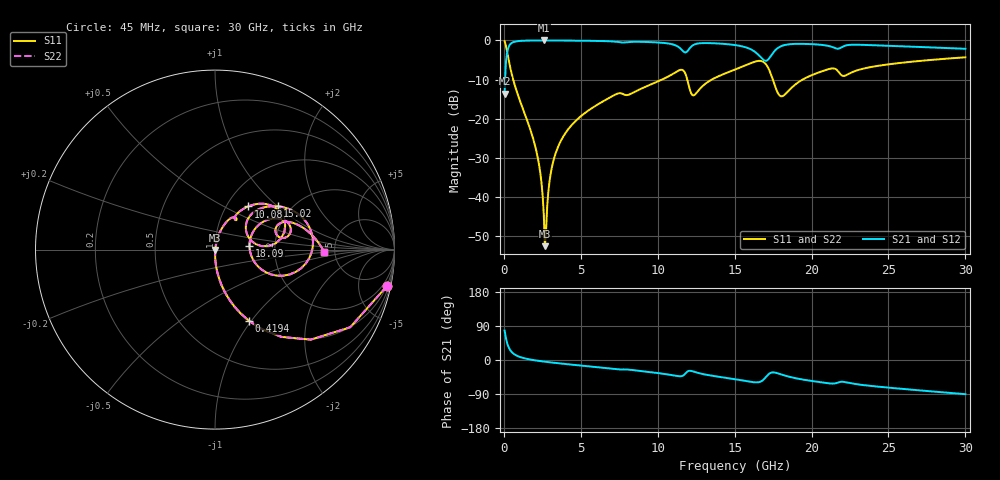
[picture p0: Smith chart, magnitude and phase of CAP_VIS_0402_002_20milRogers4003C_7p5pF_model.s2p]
! S-parameter model data by Modelithics Inc.  support@modelithics.com  813-866-6335  Tampa FL USA
! S-Parameter data specifications:
! Substrate: 20-mil Rogers 4003C, substrate thickness, H=0.508mm, Dielectric constant, Er=3.75
! PCB Mounting Pad Footprint: Pad width, PadW=0.50mm , Pad length, PadL=0.50mm , Pad gap, PadG (edge-to-edge)=0.40mm , Reference planes=1.4mm apart
! Created Wed Nov 18 12:49:41 2015
# hz S ma R 50
! 2 Port Network Data from SP1.SP block
! freq  magS11  angS11  magS21  angS21  magS12  angS12  magS22  angS22
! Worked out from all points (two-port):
!   401 points, 45 MHz to 30 GHz, reference 50 ohm
!   highest |S21| = -0.02 dB at 2.591 GHz (marker M1); lowest = -13.6 dB at 45 MHz (marker M2)
!   |S21| within 3 dB of the highest: 213.5 MHz to 11.73 GHz (11.52 GHz wide, 193 % of centre); 17.53 GHz to end of sweep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
!   lowest |S11| = -52.6 dB at 2.666 GHz (marker M3), VSWR 1.00, Z = 50.2 - j0.135 ohm
!   |S11| at or under -10 dB: 601 MHz to 10.28 GHz (9.682 GHz wide, 178 % of centre); 11.92 GHz to 13.52 GHz (1.603 GHz wide, 12.6 % of centre); 17.48 GHz to 19.43 GHz (1.946 GHz wide, 10.5 % of centre)
!   |S22| runs from -52.6 to -0.2 dB; largest |S21 - S12| = 0
!   S11 on the Smith chart (normalised r, x): 45 MHz: 0.99, -9.31; 419.4 MHz: 0.99, -0.97; 10.08 GHz: 1.26, +0.67; 15.02 GHz: 1.70, +1.00; 18.09 GHz: 1.47, +0.07; 30 GHz: 4.10, -0.17
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4.5e7  0.9779 -12.1  0.2089 77.9  0.2089 77.9  0.9779 -12.1
2.696625e8  0.6117 -52.7  0.7905 37.3  0.7905 37.3  0.6117 -52.7
4.194375e8  0.44 -64.5  0.8972 25.4  0.8972 25.4  0.44 -64.5
8.687625e8  0.2122 -78.9  0.976 10.8  0.976 10.8  0.2122 -78.9
2.066962e9  0.04177 -88.7  0.9973 -1.1  0.9973 -1.1  0.04177 -88.7
2.366512e9  0.02014 -87.5  0.9978 -2.9  0.9978 -2.9  0.02014 -87.5
2.591175e9  0.006033 -74.7  0.9979 -4.1  0.9979 -4.1  0.006033 -74.7
2.666062e9  0.00235 -34.8  0.9979 -4.5  0.9979 -4.5  0.00235 -34.8
2.815838e9  0.007757 69.2  0.9978 -5.2  0.9978 -5.2  0.007757 69.2
3.0405e9  0.01983 77.4  0.9975 -6.3  0.9975 -6.3  0.01983 77.4
3.414938e9  0.03864 78.5  0.9968 -8.0  0.9968 -8.0  0.03864 78.5
5.062462e9  0.1098 73.4  0.9907 -14.9  0.9907 -14.9  0.1098 73.4
1.007992e10  0.3033 52.4  0.9383 -34.8  0.9383 -34.8  0.3033 52.4
1.157768e10  0.4208 23.6  0.7517 -42.4  0.7517 -42.4  0.4208 23.6
1.232655e10  0.1979 25.5  0.8753 -30.5  0.8753 -30.5  0.1979 25.5
1.50225e10  0.424 34.7  0.8713 -50.7  0.8713 -50.7  0.424 34.7
1.68198e10  0.5376 -1.9  0.5739 -53.8  0.5739 -53.8  0.5376 -1.9
1.734401e10  0.3755 -22.7  0.6284 -33.8  0.6284 -33.8  0.3755 -22.7
1.809289e10  0.1934 6.6  0.8543 -38.9  0.8543 -38.9  0.1934 6.6
2.003996e10  0.3615 28.5  0.8945 -55.5  0.8945 -55.5  0.3615 28.5
2.505742e10  0.496 15.1  0.8522 -73.2  0.8522 -73.2  0.496 15.1
3e10  0.6084 -1.2  0.7811 -90.2  0.7811 -90.2  0.6084 -1.2
